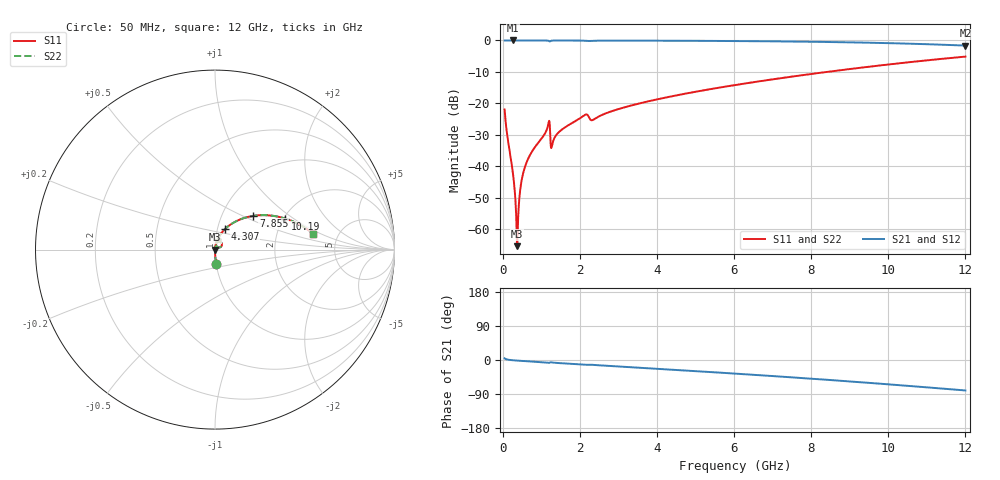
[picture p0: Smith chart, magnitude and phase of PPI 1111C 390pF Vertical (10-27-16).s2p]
# GHz S MA R 50
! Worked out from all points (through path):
!   1601 points, 50 MHz to 12 GHz, reference 50 ohm
!   highest |S21| = 0.00 dB at 259.1 MHz (marker M1); lowest = -1.6 dB at 12 GHz (marker M2)
!   group delay of S21, straight-line fit = 18.5 ps
!   lowest |S11| = -65.4 dB at 378.6 MHz (marker M3), VSWR 1.00, Z = 50.1 + j0.0135 ohm
!   |S11| at or under -10 dB: start of sweep to 8.415 GHz
!   |S22| runs from -65.4 to -5.1 dB; largest |S21 - S12| = 0
!   S11 on the Smith chart (normalised r, x): 50 MHz: 1.00, -0.16; 4.307 GHz: 1.09, +0.25; 7.855 GHz: 1.41, +0.58; 10.19 GHz: 2.04, +0.86; 12 GHz: 3.24, +0.83
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0.05  0.07983 -85.4  0.9966 4.4  0.9966 4.4  0.07983 -85.4
0.259125  0.008293 -87.5  0.9995 -0.6  0.9995 -0.6  0.008293 -87.5
0.3338125  0.002645 -80.6  0.9995 -1.2  0.9995 -1.2  0.002645 -80.6
0.378625  0.0005354 14.6  0.9995 -1.6  0.9995 -1.6  0.0005354 14.6
0.4159687  0.002271 74.5  0.9994 -1.9  0.9994 -1.9  0.002271 74.5
0.4607812  0.004511 80.7  0.9994 -2.2  0.9994 -2.2  0.004511 80.7
0.498125  0.00627 82.3  0.9994 -2.4  0.9994 -2.4  0.00627 82.3
0.5952188  0.0105 83.5  0.9993 -3.1  0.9993 -3.1  0.0105 83.5
1.162844  0.04151 75.4  0.9937 -7.2  0.9937 -7.2  0.04151 75.4
1.297281  0.02369 73.3  0.9955 -6.8  0.9955 -6.8  0.02369 73.3
1.491469  0.03638 79.6  0.9979 -8.3  0.9979 -8.3  0.03638 79.6
2.044156  0.06007 74.5  0.9944 -12.0  0.9944 -12.0  0.06007 74.5
2.163656  0.06663 66.9  0.9857 -12.8  0.9857 -12.8  0.06663 66.9
2.335437  0.0543 67.9  0.9896 -12.8  0.9896 -12.8  0.0543 67.9
4.038312  0.1168 65.8  0.9913 -23.4  0.9913 -23.4  0.1168 65.8
4.307188  0.1265 64.2  0.99 -25.0  0.99 -25.0  0.1265 64.2
6.025  0.1952 53.5  0.9784 -35.9  0.9784 -35.9  0.1952 53.5
7.854844  0.2849 41.3  0.9557 -48.3  0.9557 -48.3  0.2849 41.3
8.019156  0.2939 40.1  0.9529 -49.4  0.9529 -49.4  0.2939 40.1
10.01331  0.4153 25.3  0.9061 -64.3  0.9061 -64.3  0.4153 25.3
10.19256  0.4272 23.9  0.9005 -65.7  0.9005 -65.7  0.4272 23.9
12  0.5533 9.2  0.8286 -80.4  0.8286 -80.4  0.5533 9.2
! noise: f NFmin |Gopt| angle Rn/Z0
0.05  0.0003432  0.8556  0.265  0.0005076
1.372  0.004986  0.7441  5.648  0.003903
2.701  0.00748  0.6786  10.92  0.004458
4.031  0.00811  0.586  15.67  0.003515
5.36  0.009936  0.5631  20.33  0.003975
6.682  0.01189  0.5547  24.8  0.004575
8.012  0.01398  0.5555  29.12  0.005307
9.341  0.01628  0.5636  33.31  0.006209
10.67  0.01886  0.5781  37.4  0.007346
12  0.02181  0.5981  41.43  0.008816
